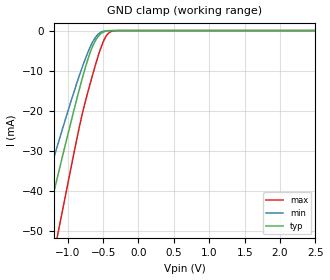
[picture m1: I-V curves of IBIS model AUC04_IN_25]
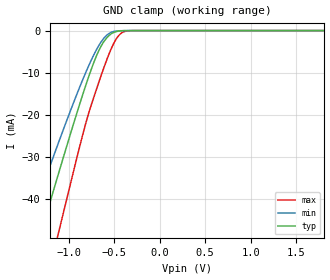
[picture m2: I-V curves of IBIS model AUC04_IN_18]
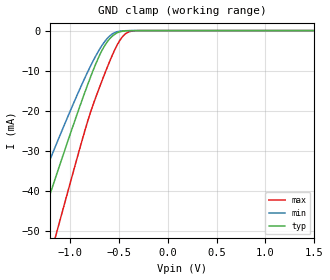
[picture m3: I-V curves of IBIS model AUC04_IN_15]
| TEXAS INSTRUMENTS INCORPORATED
| Standard Linear and Logic Group
| IBIS Model of SN74AUC04
| Hex Inverter
| This file contains package information for the following:
|  QFN 14-pin (RGY) package as [Component] AUC04_RGY
| This device can be powered at the following Vccs:
|  2.5 volt Vcc
|  1.8 volt Vcc
|  1.5 volt Vcc
|  1.2 volt Vcc
|  0.8 volt Vcc
| This file provides unique models under the [Model Selector] for each Vcc.
| For operation at a specific Vcc, select the appropriate model after each
| [Model Selector] keyword.
[IBIS Ver]   3.2
[Comment char]  |_char
[File Name]   sn74auc04.ibs
[File Rev]   1.1 | x_die
[Date]   September 25, 2002
[Source]   Data created from TI-SPICE simulations at TI-SLL.
[Notes]   The following is an IBIS list for the AUC04.
   Please contact sllibis@ti.com with questions and
   comments concerning SLL IBIS models.
   - The waveforms for the AUC04_OUT Pullup, and
   Pulldown are caused by the circuitry that helps reduce
   overshoot and undershoot in transmission lines (EMI).
   These waveforms are normal for this particular design.
   - C_comp values have been replaced by the data sheet values.
   - Power clamp data deleted as there is no power-clamp diode.
[Disclaimer] Property of Texas Instruments Incorporated.  Unauthorized
   reproduction and/or distribution is strictly prohibited.
   This product is protected under copyright law.
   Created  2002, (C) Copyright  2002, Texas Instruments
   Incorporated, All Rights Reserved
   UNLESS THERE IS A SIGNED, WRITTEN AGREEMENT TO THE
   CONTRARY, TEXAS INSTRUMENTS (TI) IS PROVIDING THE IBIS
   MODELS  AND WITHOUT ANY WARRANTY, EXPRESSED OR
   IMPLIED.  TI assumes no liability for:
   1) the accuracy of the IBIS models provided to your
   company;
   2) the proper functioning of these IBIS Models in your
   design or for any resulting applications; or
   3) infringement of patents, copyrights or intellectual
   property rights resulting from your use of these IBIS
   models.
   TI provides IBIS Models as a service to our customers.
   You and your company shall not distribute, sell or give
   these models to anyone else without prior written
   permission from TI.
   TI reserves the right to make changes to our products or
   to discontinue any semiconductor product or service
   without notice, and advises our customers to obtain the
   latest version of relevant information to verify, before
   placing orders, that the information being relied on is
   current.
   Please be aware that your receipt and use of the IBIS
   information provided shall serve as acceptance of these
   terms and conditions.  If you do not accept these terms,
   you should return or destroy the IBIS models and any
   other accompanying information immediately.
| Component AUC04_RGY 14-pin QFN
[Component]   AUC04_RGY
[Manufacturer]   Texas Instruments, Inc.
[Package]
|   typ   min   max
R_pkg   2.900e-02   2.300e-02   4.100e-02
L_pkg   7.730e-10   6.570e-10   9.980e-10
C_pkg   1.360e-13   1.150e-13   1.560e-13
[Pin]   signal_name   model_name   R_pin   L_pin   C_pin
1   1A   AUC04_IN   2.700e-02   8.310e-10   1.300e-13
2   1Y   AUC04_OUT   2.700e-02   8.660e-10   1.350e-13
3   2A   AUC04_IN   4.100e-02   9.980e-10   1.560e-13
4   2Y   AUC04_OUT   3.100e-02   7.670e-10   1.420e-13
5   3A   AUC04_IN   3.100e-02   7.650e-10   1.420e-13
6   3Y   AUC04_OUT   3.100e-02   7.830e-10   1.440e-13
7   GND   GND   3.100e-02   7.810e-10   1.370e-13
8   4Y   AUC04_OUT   2.300e-02   6.570e-10   1.150e-13
9   4A   AUC04_IN   2.300e-02   8.140e-10   1.290e-13
10   5Y   AUC04_OUT   2.800e-02   7.040e-10   1.290e-13
11   5A   AUC04_IN   2.700e-02   6.720e-10   1.360e-13
12   6Y   AUC04_OUT   2.700e-02   6.960e-10   1.380e-13
13   6A   AUC04_IN   2.700e-02   7.250e-10   1.400e-13
14   VCC   POWER   3.000e-02   7.630e-10   1.360e-13
| Model AUC04_IN
[Model Selector]   AUC04_IN
AUC04_IN_25   2.5 volt Vcc
AUC04_IN_18   1.8 volt Vcc
AUC04_IN_15   1.5 volt Vcc
AUC04_IN_12   1.2 volt Vcc
AUC04_IN_08   0.8 volt Vcc
| Model AUC04_OUT
[Model Selector]   AUC04_OUT
AUC04_OUT_25   2.5 volt Vcc
AUC04_OUT_18   1.8 volt Vcc
AUC04_OUT_15   1.5 volt Vcc
AUC04_OUT_12   1.2 volt Vcc
AUC04_OUT_08   0.8 volt Vcc
| Models and submodels in the file (10): AUC04_IN_25 (Input), AUC04_IN_18 (Input), AUC04_IN_15 (Input), AUC04_IN_12 (Input), AUC04_IN_08 (Input), AUC04_OUT_25 (Output), AUC04_OUT_18 (Output), AUC04_OUT_15 (Output), AUC04_OUT_12 (Output), AUC04_OUT_08 (Output)
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[Model]   AUC04_IN_25
Model_type  Input
Vinl=0.7
Vinh=1.7
| variable   typ   min   max
C_comp   2.29pF   1.82pF   2.66pF
[Temperature Range]   40   100   -40
| Ambient temperature   25   85   -40
[Voltage range]   2.5   2.3   2.7
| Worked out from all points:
|   GND clamp passes 1 mA (typ) near -0.55 V on its own axis
[GND Clamp]
| AUC04_IN_25
|   Voltage   I(typ)   I(min)   I(max)
-3.6V     -222.3mA   -186.1mA   -267.5mA
-1.49V    -62.29mA   -49.79mA   -82.1mA
-1.35V    -51.8mA    -41.14mA   -69.63mA
-1.305V   -48.45mA   -38.39mA   -65.61mA
-1.17V    -38.46mA   -30.25mA   -53.55mA
-1.12V    -34.79mA   -27.28mA   -49.08mA
-735mV    -8.324mA   -6.331mA   -16.67mA
-635mV    -3.426mA   -2.471mA   -10.25mA
-525mV    -682.5uA   -360.4uA   -4.021mA
-430mV    -73.19uA   -34.73uA   -776.9uA
-325mV    -3.339uA   -2.006uA   -30.74uA
2.5V      313.9pA    400.9pA    470.4pA
[Model]   AUC04_IN_18
Model_type  Input
Vinl=0.5775
Vinh=1.2675
| variable   typ   min   max
C_comp   2.36pF   1.92pF   2.68pF
[Temperature Range]   40   100   -40
| Ambient temperature   25   85   -40
[Voltage range]   1.8   1.65   1.95
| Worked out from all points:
|   GND clamp passes 1 mA (typ) near -0.55 V on its own axis
[GND Clamp]
| AUC04_IN_18
|   Voltage   I(typ)   I(min)   I(max)
-3.6V     -222.3mA   -186.1mA   -267.5mA
-1.475V   -61.16mA   -48.85mA   -80.77mA
-1.43V    -57.79mA   -46.07mA   -76.76mA
-1.295V   -47.7mA    -37.79mA   -64.71mA
-1.145V   -36.62mA   -28.76mA   -51.31mA
-1.095V   -32.97mA   -25.81mA   -46.85mA
-830mV    -14.31mA   -10.96mA   -23.64mA
-685mV    -5.607mA   -4.224mA   -13.41mA
-560mV    -1.272mA   -753.7uA   -5.827mA
-485mV    -290.6uA   -140.2uA   -2.305mA
-420mV    -55.81uA   -26.72uA   -608.5uA
1.8V      203.2pA    297.2pA    235.5pA
[Model]   AUC04_IN_15
Model_type  Input
Vinl=0.49
Vinh=1.04
| variable   typ   min   max
C_comp   2.39pF   1.97pF   2.74pF
[Temperature Range]   40   100   -40
| Ambient temperature   25   85   -40
[Voltage range]   1.5   1.4   1.6
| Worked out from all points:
|   GND clamp passes 1 mA (typ) near -0.55 V on its own axis
[GND Clamp]
| AUC04_IN_15
|   Voltage   I(typ)   I(min)   I(max)
-3.6V     -222.3mA   -186.1mA   -267.5mA
-1.505V   -63.42mA   -50.72mA   -83.44mA
-1.325V   -49.94mA   -39.61mA   -67.39mA
-1.17V    -38.46mA   -30.25mA   -53.55mA
-1.12V    -34.79mA   -27.28mA   -49.08mA
-840mV    -14.98mA   -11.48mA   -24.46mA
-695mV    -6.114mA   -4.621mA   -14.06mA
-570mV    -1.487mA   -911.6uA   -6.381mA
-495mV    -364.6uA   -178.8uA   -2.692mA
-430mV    -73.19uA   -34.73uA   -776.9uA
-280mV    -781.4nA   -556.3nA   -5.358uA
1.5V      165.9pA    258.5pA    172.1pA
